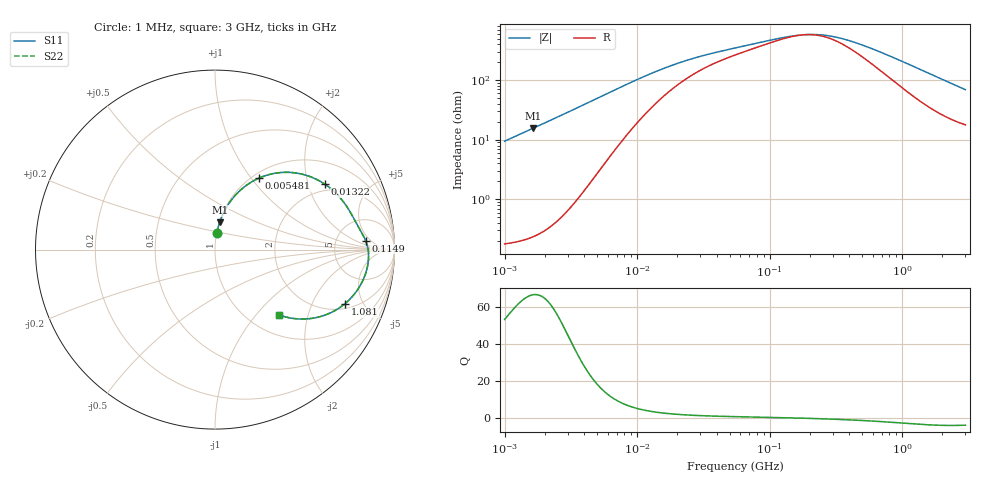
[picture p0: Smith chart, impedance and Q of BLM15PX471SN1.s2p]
! BLM15PX471SN1
# Hz S RI R 50
!Freq.(Hz) S11(Real) S11(Imag) S21(Real) S21(Imag) S12(Real) S12(Imag) S22(Real) S22(Imag)
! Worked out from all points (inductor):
!   401 points, 1 MHz to 3 GHz, reference 50 ohm
!   read as one part in series: L = 1.51 uH near 1.041 MHz
!   highest Q = 66.3 at 1.649 MHz (marker M1), where L = 1.51 uH
!   self-resonance near 183.5 MHz
!   S11 on the Smith chart (normalised r, x): 1 MHz: 1.00, +0.19; 5.481 MHz: 1.07, +1.09; 13.22 MHz: 1.74, +2.58; 114.9 MHz: 10, +4; 1.081 GHz: 2.30, -3.61; 3 GHz: 1.36, -1.34
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1000000  0.0106 0.0933  0.9894 -0.0933  0.9894 -0.0933  0.0106 0.0933
1649378  0.0262 0.1522  0.9738 -0.1522  0.9738 -0.1522  0.0262 0.1522
2613693  0.0632 0.2341  0.9368 -0.2341  0.9368 -0.2341  0.0632 0.2341
3823119  0.1304 0.3206  0.8696 -0.3206  0.8696 -0.3206  0.1304 0.3206
5481359  0.2445 0.3983  0.7555 -0.3983  0.7555 -0.3983  0.2445 0.3983
6831390  0.3382 0.426  0.6618 -0.426  0.6618 -0.426  0.3382 0.426
8345207  0.4302 0.4292  0.5698 -0.4292  0.5698 -0.4292  0.4302 0.4292
1.322427e7  0.6125 0.3642  0.3875 -0.3642  0.3875 -0.3642  0.6125 0.3642
1.461624e7  0.6416 0.3427  0.3584 -0.3427  0.3584 -0.3427  0.6416 0.3427
2.459509e7  0.7387 0.2332  0.2613 -0.2332  0.2613 -0.2332  0.7387 0.2332
5.477226e7  0.8011 0.1226  0.1989 -0.1226  0.1989 -0.1226  0.8011 0.1226
1.148668e8  0.8391 0.0505  0.1609 -0.0505  0.1609 -0.0505  0.8391 0.0505
1.614254e8  0.8504 0.0145  0.1496 -0.0145  0.1496 -0.0145  0.8504 0.0145
2.094008e8  0.8549 -0.0156  0.1451 0.0156  0.1451 0.0156  0.8549 -0.0156
2.716345e8  0.8554 -0.0485  0.1446 0.0485  0.1446 0.0485  0.8554 -0.0485
3.594878e8  0.8507 -0.0883  0.1493 0.0883  0.1493 0.0883  0.8507 -0.0883
5.583748e8  0.8277 -0.1632  0.1723 0.1632  0.1723 0.1632  0.8277 -0.1632
8.005644e8  0.7851 -0.2368  0.2149 0.2368  0.2149 0.2368  0.7851 -0.2368
1.080907e9  0.7238 -0.3016  0.2762 0.3016  0.2762 0.3016  0.7238 -0.3016
1.855641e9  0.544 -0.3825  0.456 0.3825  0.456 0.3825  0.544 -0.3825
2.312676e9  0.4563 -0.3858  0.5437 0.3858  0.5437 0.3858  0.4563 -0.3858
3e9  0.3583 -0.3645  0.6417 0.3645  0.6417 0.3645  0.3583 -0.3645
